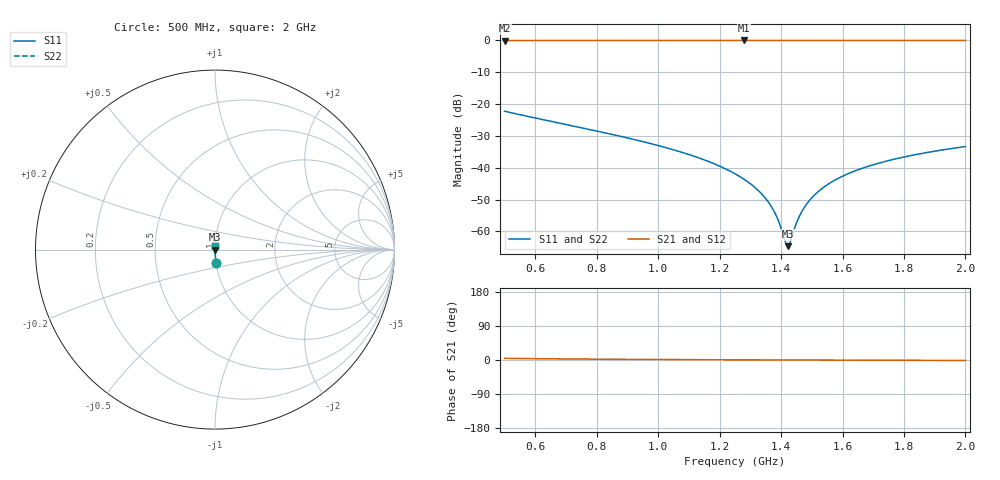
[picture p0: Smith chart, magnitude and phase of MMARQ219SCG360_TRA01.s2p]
! MMARQ219SCG360_TRA01  S-PARAMETER MODEL  ( General Type )
! Model Generated by TAIYO YUDEN Corporation (http://www.ty-top.com)
! Version 1.0
! TAIYO YUDEN Control No. 180601
! Copyright(c) 2018 TAIYO YUDEN CO.,LTD. All Rights Reserved.
! Product Description (link to TY-COMPAS)
! https://ds.yuden.co.jp/TYCOMPAS/or/detail?pn=MMARQ219SCG360JTRA01&u=M
! Products Name : Multilayer Ceramic Capacitors
! Characteristics :
!  Capacitance : 36 pF , Rated Voltage : 250V , TCC : CG / C0G
!  Case Size : 2.0 x 1.25 / 0.079 x 0.049 [mm/inch] , Thickness : 0.85 / 0.033 [mm/inch]
!  (Conditions: Temperature = 25 degC , DC Bias Current/Voltage = 0A / 0V)
! External Node Assignments :
!  1  o---| |---o  2
! GND o---------o GND
! Frequency Range : 500MHz  -  2000MHz  [ 401 STEP ]
# MHz S RI R 50
! Freq[MHz].  S11 Real  S11 Imag  S21 Real  S21 Imag  S12 Real  S12 Imag  S22 Real  S22 Imag
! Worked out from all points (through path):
!   401 points, 500 MHz to 2 GHz, reference 50 ohm
!   highest |S21| = 0.00 dB at 1.28 GHz (marker M1); lowest = 0.0 dB at 500 MHz (marker M2)
!   lowest |S11| = -64.7 dB at 1.423 GHz (marker M3), VSWR 1.00, Z = 50.1 + j0.00227 ohm
!   |S11| at or under -10 dB: start of sweep to end of sweep
!   |S22| runs from -64.7 to -22.3 dB; largest |S21 - S12| = 0
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500  0.0063 -0.0769  0.9937 0.0769  0.9937 0.0769  0.0063 -0.0769
751.25  0.00219 -0.0423  0.9978 0.0423  0.9978 0.0423  0.00219 -0.0423
1002.5  0.000946 -0.0221  0.9991 0.0221  0.9991 0.0221  0.000946 -0.0221
1145  0.00068 -0.0135  0.9993 0.0135  0.9993 0.0135  0.00068 -0.0135
1250  0.000593 -0.00801  0.9994 0.00801  0.9994 0.00801  0.000593 -0.00801
1280  0.00058 -0.00653  0.9994 0.00653  0.9994 0.00653  0.00058 -0.00653
1325  0.000571 -0.00438  0.9994 0.00438  0.9994 0.00438  0.000571 -0.00438
1362.5  0.000571 -0.00265  0.9994 0.00265  0.9994 0.00265  0.000571 -0.00265
1388.75  0.000575 -0.00146  0.9994 0.00146  0.9994 0.00146  0.000575 -0.00146
1415  0.000581 -0.000305  0.9994 0.000305  0.9994 0.000305  0.000581 -0.000305
1422.5  0.000584 2.27e-05  0.9994 -2.27e-05  0.9994 -2.27e-05  0.000584 2.27e-05
1430  0.000586 0.000348  0.9994 -0.000348  0.9994 -0.000348  0.000586 0.000348
1448.75  0.000594 0.00115  0.9994 -0.00115  0.9994 -0.00115  0.000594 0.00115
1463.75  0.000601 0.00179  0.9994 -0.00179  0.9994 -0.00179  0.000601 0.00179
1482.5  0.000611 0.00258  0.9994 -0.00258  0.9994 -0.00258  0.000611 0.00258
1501.25  0.000622 0.00336  0.9994 -0.00336  0.9994 -0.00336  0.000622 0.00336
1542.5  0.00065 0.00504  0.9994 -0.00504  0.9994 -0.00504  0.00065 0.00504
1598.75  0.000697 0.00726  0.9993 -0.00726  0.9993 -0.00726  0.000697 0.00726
1666.25  0.000765 0.00984  0.9992 -0.00984  0.9992 -0.00984  0.000765 0.00984
1752.5  0.000868 0.013  0.9991 -0.013  0.9991 -0.013  0.000868 0.013
1868.75  0.00103 0.0171  0.999 -0.0171  0.999 -0.0171  0.00103 0.0171
2000  0.00125 0.0215  0.9988 -0.0215  0.9988 -0.0215  0.00125 0.0215
